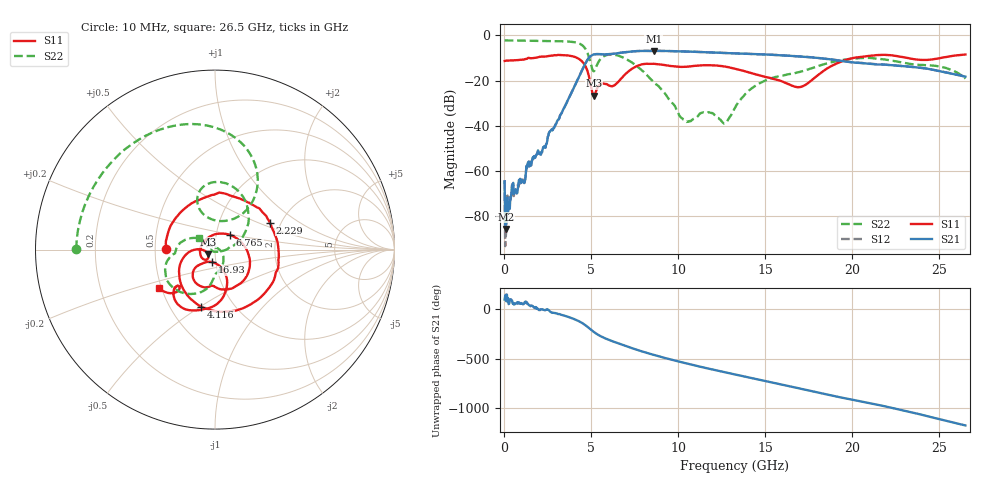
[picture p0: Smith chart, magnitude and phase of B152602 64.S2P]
!  2-Port S-parameters saved by WinCal
! VAR MeasName=S-Parameters (CALIBRATED_DATA) read from VNA (N5242A)
! VAR MeasDate=2016-1-5 16:34:49
! VAR NAME=B152602 64
! VAR FILENAME=B152602 64.S2P
! VAR DATE=2016-1-5 16:34:49
! VAR PHYS_PORTS=1,2
# Hz S DB R 50
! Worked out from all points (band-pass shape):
!   801 points, 10 MHz to 26.5 GHz, reference 50 ohm
!   highest |S21| = -6.85 dB at 8.586 GHz (marker M1); lowest = -85.6 dB at 76.22 MHz (marker M2)
!   |S21| within 3 dB of the highest: 4.868 GHz to 17.84 GHz (12.97 GHz wide, 114 % of centre)
!   lowest |S11| = -26.7 dB at 5.142 GHz (marker M3), VSWR 1.10, Z = 46.2 - j2.27 ohm
!   |S11| at or under -10 dB: start of sweep to 1.356 GHz; 4.188 GHz to 20.05 GHz (15.86 GHz wide, 131 % of centre); 23.19 GHz to 25.08 GHz (1.889 GHz wide, 7.83 % of centre)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
!   |S22| runs from -39.0 to -2.2 dB; largest |S21 - S12| = 0.0032
!   S11 on the Smith chart (normalised r, x): 10 MHz: 0.57, +0.00; 2.229 GHz: 1.75, +0.59; 4.116 GHz: 0.71, -0.50; 6.765 GHz: 1.17, +0.19; 16.93 GHz: 0.96, -0.14; 26.5 GHz: 0.49, -0.25
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1e7  -11.30 179.4  -64.58 92.6  -63.99 109.2  -2.24 179.8
7.6225e7  -11.23 175.2  -85.63 141.7  -89.27 -52.3  -2.24 178.8
1.755625e8  -11.15 167.9  -71.80 75.4  -70.83 91.3  -2.24 177.3
4.73575e8  -11.05 146.6  -65.77 52.8  -66.87 63.6  -2.26 172.7
2.228538e9  -9.38 26.2  -49.42 -7.9  -49.46 -7.3  -2.41 144.2
4.11595e9  -9.71 -104.1  -21.04 -111.0  -21.04 -111.0  -3.16 94.6
4.447075e9  -11.38 -134.7  -15.57 -140.7  -15.55 -140.7  -4.21 76.7
5.142438e9  -26.70 -148.0  -8.43 127.0  -8.42 127.0  -15.85 86.5
5.804688e9  -21.46 -171.0  -8.38 62.3  -8.37 62.3  -8.87 99.5
6.76495e9  -18.69 43.8  -7.60 -1.0  -7.60 -0.9  -9.57 61.7
8.586138e9  -12.54 -66.8  -6.85 -103.1  -6.85 -103.0  -20.78 10.1
8.851038e9  -12.79 -74.5  -6.87 -116.1  -6.84 -116.2  -22.39 5.8
1.044044e10  -13.87 -96.0  -7.13 172.0  -7.11 172.2  -38.14 -78.3
1.16656e10  -13.19 -110.6  -7.52 121.6  -7.49 121.7  -34.22 174.9
1.269209e10  -13.82 -126.0  -7.79 81.8  -7.79 81.7  -38.80 70.1
1.3255e10  -14.74 -132.2  -7.95 60.4  -7.93 60.3  -32.00 -0.9
1.45795e10  -17.49 -137.4  -8.30 10.1  -8.30 10.1  -21.49 -56.7
1.693049e10  -22.93 -101.4  -9.28 -79.0  -9.30 -78.9  -16.24 -92.4
1.769208e10  -19.62 -71.3  -9.73 -108.3  -9.71 -108.0  -14.48 -96.4
1.951326e10  -11.15 -82.0  -11.44 -176.7  -11.40 -176.5  -10.79 -121.5
2.209604e10  -8.68 -124.5  -13.10 91.6  -13.02 91.2  -10.94 -163.9
2.65e10  -8.44 -145.1  -18.24 -91.8  -18.23 -92.1  -19.11 145.8
